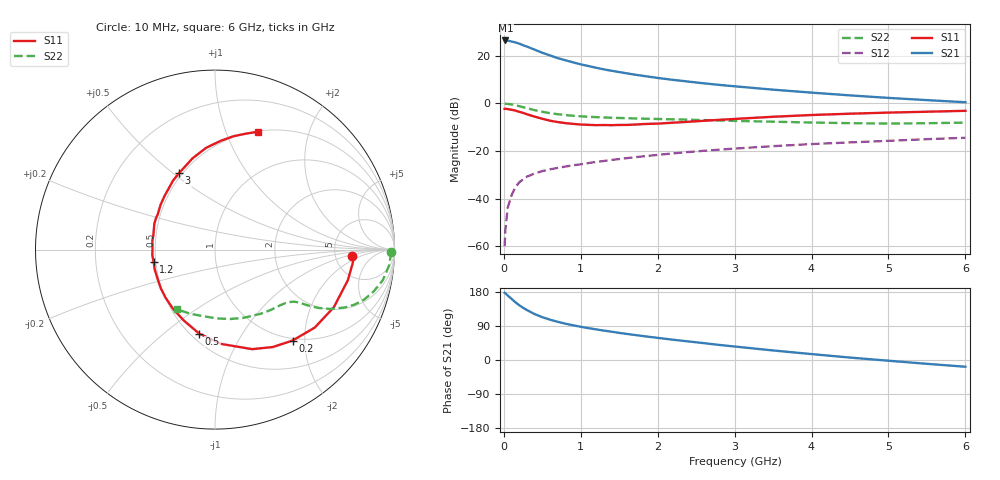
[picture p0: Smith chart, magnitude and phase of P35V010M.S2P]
! SIEMENS Small Signal Semiconductors
! BFP181
! Si NPN RF Bipolar Junction Transistor in SOT143
! VCE = 5 V  IC = 10 mA
! Common Emitter S-Parameters:  March  1996
# GHz  S  MA  R  50
!  f  S11  S21  S12  S22
! GHz  MAG  ANG  MAG  ANG  MAG  ANG  MAG  ANG
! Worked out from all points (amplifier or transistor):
!   36 points, 10 MHz to 6 GHz, reference 50 ohm
!   highest |S21| = 26.4 dB at 20 MHz (marker M1)
!   |S21| within 3 dB of that: start of sweep to 332.9 MHz
!   unconditionally stable (mu >= 1): 1.244 GHz to end of sweep
!   at 250 MHz: K = 0.32, MSG = 28.2 dB, |S12| = -32.0 dB
!   at 1.4 GHz: K = 1.04, MAG = 17.5 dB, |S12| = -23.8 dB
!   at 6 GHz: K = 1.02, MAG = 6.7 dB, |S12| = -14.5 dB
!   S11 on the Smith chart (normalised r, x): 10 MHz: 7.33, -1.28; 200 MHz: 0.96, -1.75; 500 MHz: 0.55, -0.67; 1.2 GHz: 0.49, -0.08; 3 GHz: 0.48, +0.53; 6 GHz: 0.51, +1.30
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0.01  0.7664 -2.7  20.94 177.5  0.001 71.5  0.9807 -0.8
0.02  0.7721 -5.2  21 176.1  0.0022 91.8  0.9795 -2.0
0.05  0.7597 -12.9  20.8 170.3  0.0064 86.8  0.9741 -5.2
0.1  0.736 -25.8  19.92 161.3  0.0117 75.7  0.9506 -10.3
0.15  0.7055 -38.0  19.11 152.4  0.0173 71.0  0.9149 -14.7
0.2  0.6661 -49.5  18.01 144.6  0.022 66.9  0.8747 -18.7
0.25  0.6313 -59.3  16.69 137.8  0.0252 63.1  0.8326 -21.7
0.3  0.5922 -69.5  15.62 131.9  0.0289 59.5  0.7926 -24.0
0.4  0.5267 -86.3  13.44 121.1  0.0337 55.7  0.7206 -27.3
0.5  0.4758 -100.7  11.56 113.0  0.0377 52.1  0.6652 -29.3
0.6  0.4325 -113.4  10.18 106.4  0.0412 50.3  0.6239 -30.5
0.7  0.4055 -124.9  8.932 100.8  0.0441 49.7  0.5922 -31.3
0.8  0.3847 -135.6  8.059 95.8  0.0471 49.2  0.568 -31.8
1.1  0.3539 -161.3  6.093 84.0  0.0558 49.0  0.5232 -33.7
1.2  0.3489 -168.5  5.595 80.8  0.0589 48.5  0.5143 -34.5
1.7  0.3581 162.1  4.019 66.1  0.0738 47.9  0.4832 -39.3
2.2  0.3932 140.4  3.12 53.5  0.089 45.8  0.4618 -45.6
3  0.4708 115.1  2.285 35.6  0.1123 40.8  0.4287 -58.0
3.5  0.5234 103.9  1.942 25.2  0.1263 37.4  0.4124 -67.1
4.5  0.6072 86.9  1.473 6.4  0.1515 29.5  0.3839 -88.4
5.5  0.6679 75.2  1.171 -10.1  0.1772 22.5  0.3831 -111.0
6  0.6979 70.1  1.057 -17.8  0.1893 18.6  0.3948 -122.4
